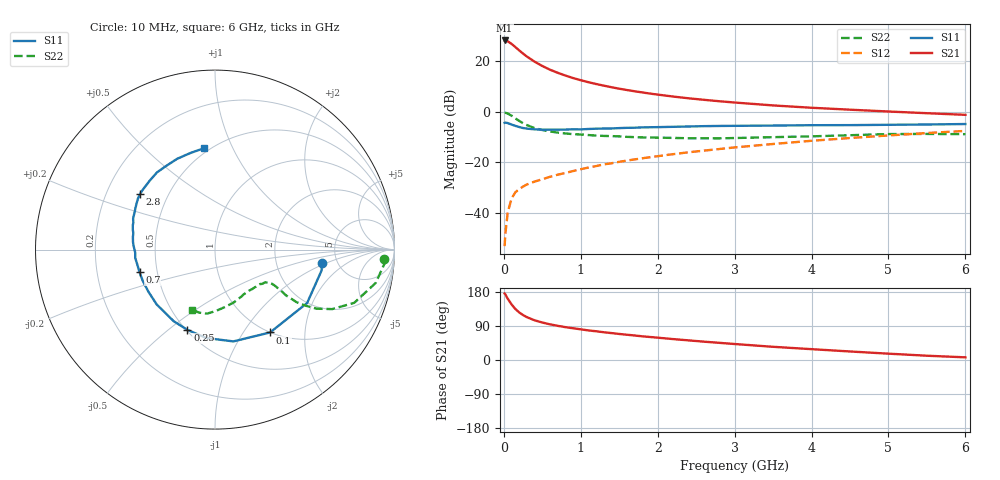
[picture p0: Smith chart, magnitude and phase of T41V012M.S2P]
! Infineon Technologies  Discrete & RF Semiconductors
! BFR182T
! Si NPN RF Bipolar Junction Transistor in SC75
! VCE = 1 V  IC = 12 mA
! Common Emitter S-Parameters:  October  1999
# GHz  S  MA  R  50
!  f  S11  S21  S12  S22
! GHz  MAG  ANG  MAG  ANG  MAG  ANG  MAG  ANG
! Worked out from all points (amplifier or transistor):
!   36 points, 10 MHz to 6 GHz, reference 50 ohm
!   highest |S21| = 28.1 dB at 10 MHz (marker M1)
!   |S21| within 3 dB of that: start of sweep to 164.7 MHz
!   unconditionally stable (mu >= 1): 627.7 MHz to 4.445 GHz
!   at 250 MHz: K = 0.59, MSG = 26.2 dB, |S12| = -29.6 dB
!   at 1.4 GHz: K = 1.21, MAG = 12.3 dB, |S12| = -20.4 dB
!   at 6 GHz: K = 0.92, MSG = 3.2 dB, |S12| = -7.6 dB
!   S11 on the Smith chart (normalised r, x): 10 MHz: 3.76, -0.89; 100 MHz: 1.00, -1.33; 250 MHz: 0.51, -0.58; 700 MHz: 0.40, -0.12; 2.8 GHz: 0.35, +0.30; 6 GHz: 0.47, +0.78
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0.01  0.599 -7.3  25.35 175.5  0.0022 83.6  0.9431 -3.2
0.02  0.6054 -11.0  25.31 172.9  0.0039 79.4  0.9472 -4.8
0.05  0.5933 -30.1  24.43 161.9  0.0101 76.1  0.9145 -11.7
0.1  0.5543 -56.4  21.71 146.8  0.0192 69.7  0.8307 -20.9
0.15  0.5216 -78.7  18.76 134.5  0.0255 61.6  0.7327 -26.9
0.2  0.495 -95.6  16.14 125.5  0.0295 58.9  0.6548 -30.2
0.25  0.4728 -109.0  13.94 118.6  0.0331 55.4  0.5877 -31.9
0.3  0.4605 -120.0  12.19 113.0  0.0364 55.6  0.5405 -32.8
0.4  0.446 -136.7  9.661 104.7  0.0415 54.8  0.4712 -32.8
0.5  0.439 -147.7  7.942 98.9  0.0461 56.9  0.432 -31.9
0.6  0.4385 -156.6  6.712 94.1  0.0515 58.0  0.4046 -31.4
0.7  0.439 -163.3  5.828 90.2  0.0567 59.7  0.3843 -31.0
0.9  0.4469 -174.0  4.591 83.7  0.0669 62.3  0.3581 -31.2
1.1  0.4531 177.8  3.8 78.0  0.0785 63.7  0.3438 -32.2
1.3  0.4629 171.1  3.249 73.2  0.0905 64.9  0.3306 -34.0
1.6  0.4775 163.5  2.662 66.7  0.1079 65.8  0.3168 -37.2
2.2  0.5 152.4  1.98 55.2  0.1442 66.1  0.3019 -46.7
2.8  0.5199 143.3  1.6 45.3  0.182 64.7  0.2962 -57.6
3.5  0.5291 133.3  1.322 34.8  0.2291 62.1  0.3123 -70.5
4.5  0.5398 120.2  1.089 22.5  0.3007 56.5  0.3411 -88.8
5.5  0.5557 104.1  0.928 11.3  0.3768 49.6  0.362 -104.1
6  0.5677 96.3  0.862 7.0  0.4155 45.3  0.3578 -110.9
